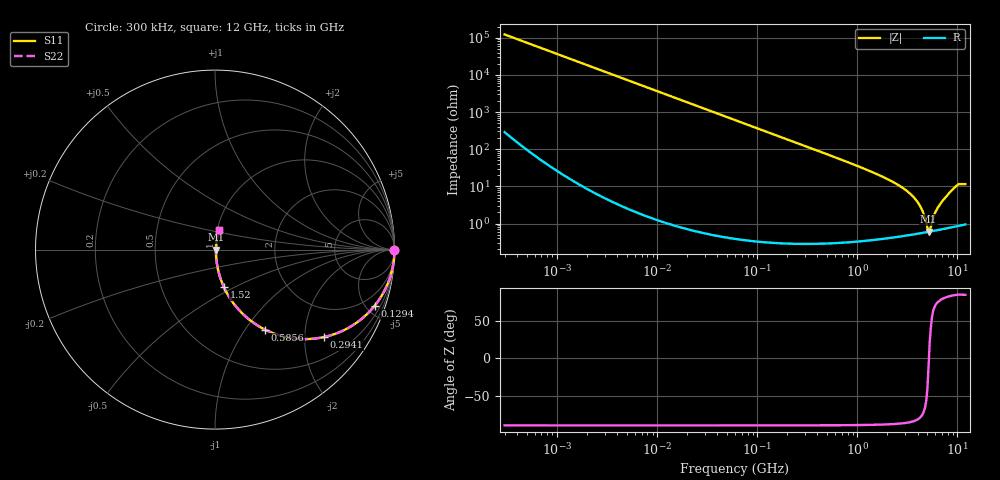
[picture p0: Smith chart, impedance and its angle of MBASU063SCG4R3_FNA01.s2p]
! MBASU063SCG4R3_FNA01  S-PARAMETER MODEL  ( Standard Model )
! Model Generated by TAIYO YUDEN Corporation (http://www.ty-top.com)
! Version 1.0
! TAIYO YUDEN Control No. 230609
! Copyright(c) 2023 TAIYO YUDEN CO.,LTD. All Rights Reserved.
! Product Description (link to TY-COMPAS)
! https://ds.yuden.co.jp/TYCOMPAS/or/detail?pn=MBASU063SCG4R3BFNA01&u=M
! Products Name : Multilayer Ceramic Capacitors
! Characteristics :
!  Capacitance : 4.3 [pF] , Rated Voltage : 50 [V] , TCC : CG / C0G
!  Case Size : 0.6 x 0.3 / 0.024 x 0.012 [mm/inch] , Thickness : 0.3 / 0.012 [mm/inch]
!  (Conditions: Temperature = 25 [degC] , DC Bias Voltage = 0 [V])
! External Node Assignments :
!  1  o---| |---o  2
! GND o---------o GND
! Frequency Range : 0.3MHz  -  12000MHz  [ 401 STEP ]
# MHZ S RI R 50
! Freq[MHz].  S11 Real  S11 Imag  S21 Real  S21 Imag  S12 Real  S12 Imag  S22 Real  S22 Imag
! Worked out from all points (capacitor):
!   401 points, 300 kHz to 12 GHz, reference 50 ohm
!   read as one part in series: C = 4.33 pF near 316.3 kHz
!   lowest |Z| = 609 mohm at 5.141 GHz (marker M1)
!   series resonance near 5.188 GHz, so ESL is about 220 pH
!   S11 on the Smith chart (normalised r, x): 300 kHz: open; 129.4 MHz: 1.01, -5.68; 294.1 MHz: 1.01, -2.49; 585.6 MHz: 1.01, -1.24; 1.52 GHz: 1.01, -0.44; 12 GHz: 1.02, +0.23
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0.3  1 -0.000815  2.57e-06 0.000815  2.57e-06 0.000815  1 -0.000815
1.769972  1 -0.00481  2.55e-05 0.00481  2.55e-05 0.00481  1 -0.00481
10.44266  0.9992 -0.0284  0.000815 0.0284  0.000815 0.0284  0.9992 -0.0284
60  0.974 -0.1588  0.026 0.1588  0.026 0.1588  0.974 -0.1588
129.3602  0.8896 -0.3129  0.1104 0.3129  0.1104 0.3129  0.8896 -0.3129
192.4766  0.7843 -0.4106  0.2157 0.4106  0.2157 0.4106  0.7843 -0.4106
294.0765  0.6084 -0.487  0.3916 0.487  0.3916 0.487  0.6084 -0.487
353.9943  0.5169 -0.4984  0.4831 0.4984  0.4831 0.4984  0.5169 -0.4984
585.5907  0.2788 -0.446  0.7212 0.446  0.7212 0.446  0.2788 -0.446
918.7169  0.1328 -0.3353  0.8672 0.3353  0.8672 0.3353  0.1328 -0.3353
1519.776  0.0498 -0.2095  0.9502 0.2095  0.9502 0.2095  0.0498 -0.2095
2088.533  0.0251 -0.1434  0.9749 0.1434  0.9749 0.1434  0.0251 -0.1434
2947.191  0.0116 -0.0832  0.9884 0.0832  0.9884 0.0832  0.0116 -0.0832
3740.715  0.00731 -0.0467  0.9927 0.0467  0.9927 0.0467  0.00731 -0.0467
4385.161  0.00606 -0.0238  0.9939 0.0238  0.9939 0.0238  0.00606 -0.0238
5006.236  0.00588 -0.00508  0.9941 0.00508  0.9941 0.00508  0.00588 -0.00508
5140.631  0.00593 -0.00119  0.9941 0.00119  0.9941 0.00119  0.00593 -0.00119
5420.343  0.00611 0.00527  0.9939 -0.00527  0.9939 -0.00527  0.00611 0.00527
6188.031  0.00699 0.0221  0.993 -0.0221  0.993 -0.0221  0.00699 0.0221
7448.838  0.00932 0.0462  0.9907 -0.0462  0.9907 -0.0462  0.00932 0.0462
9968.853  0.0196 0.1049  0.9804 -0.1049  0.9804 -0.1049  0.0196 0.1049
12000  0.022 0.1111  0.978 -0.1111  0.978 -0.1111  0.022 0.1111
